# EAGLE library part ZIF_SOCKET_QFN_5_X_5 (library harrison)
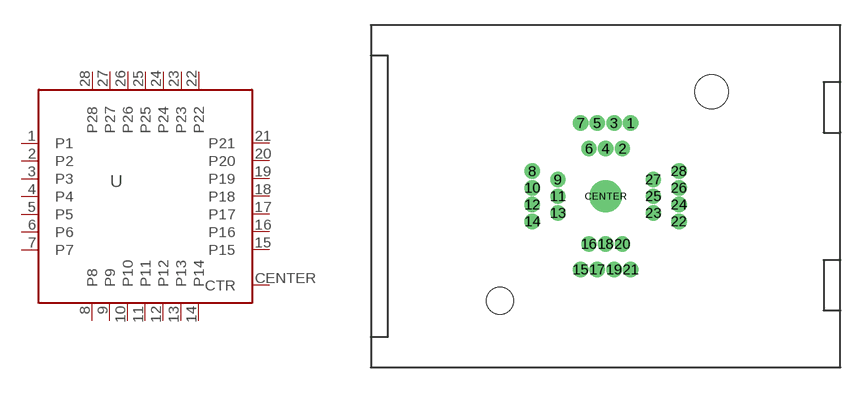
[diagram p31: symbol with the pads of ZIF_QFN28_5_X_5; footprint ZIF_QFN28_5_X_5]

Designator prefix U

## ZIF_SOCKET_QFN_5_X_5  [ZIF_QFN28_5_X_5]
1  P1
2  P2
3  P3
4  P4
5  P5
6  P6
7  P7
8  P8
9  P9
10  P10
11  P11
12  P12
13  P13
14  P14
15  P15
16  P16
17  P17
18  P18
19  P19
20  P20
21  P21
22  P22
23  P23
24  P24
25  P25
26  P26
27  P27
28  P28
CENTER  CTR

## Footprint ZIF_QFN28_5_X_5 (pad centres in mm)
drill 0.41 pad 0.813: 1 1.5,4.37; 2 1,2.845; 3 0.5,4.37; 4 0,2.845; 5 -0.5,4.37; 6 -1,2.845; 7 -1.5,4.37; 8 -4.37,1.5; 9 -2.845,1; 10 -4.37,0.5; 11 -2.845,0; 12 -4.37,-0.5; 13 -2.845,-1; 14 -4.37,-1.5; 15 -1.5,-4.37; 16 -1,-2.845; 17 -0.5,-4.37; 18 0,-2.845; 19 0.5,-4.37; 20 1,-2.845; 21 1.5,-4.37; 22 4.37,-1.5; 23 2.845,-1; 24 4.37,-0.5; 25 2.845,0; 26 4.37,0.5; 27 2.845,1; 28 4.37,1.5
drill 1.02 pad 1.93: CENTER 0,0
hole 1.6 at -6.31,-6.23
hole 2 at 6.31,6.23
